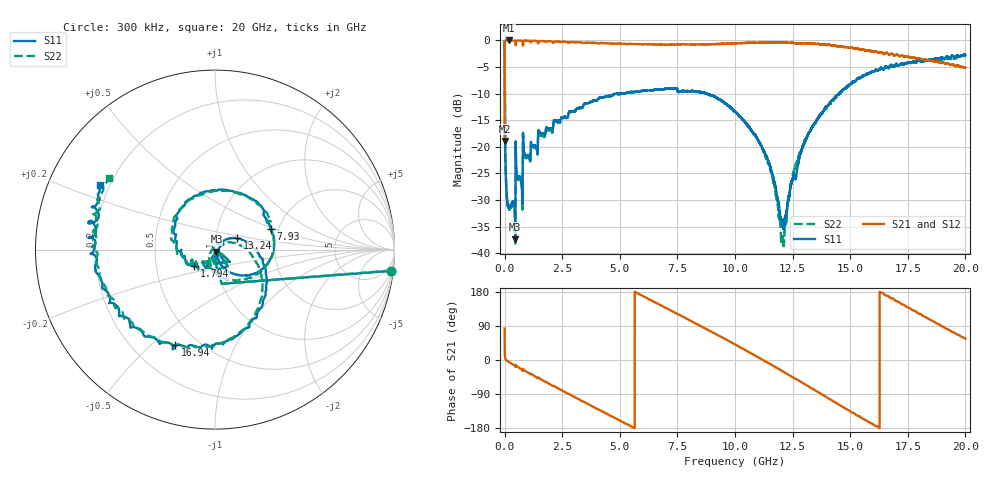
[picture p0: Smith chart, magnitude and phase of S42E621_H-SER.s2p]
!{S42E621}
!Johanson Technology Inc.
!www.johansontechnology.com
!Test Board Conditions:
!Substrate Type  RO4350B
!Substrate Thickness  50 mil
!Substrate Dk  3.66
!TL Type: GCPW
!TL Trace Width  60 mil
!TL Gap  10 mil
!Electrode orientation  Horizontal
!DUT TOPOLOGY	SERIES
!Mounting Pad LxW  14x55 mil
! Created Wed Nov 25 22:22:56 2020
# khz S ma R 50
! 2 Port Network Data from SP1.SP block
! freq  magS11  angS11  magS21  angS21  magS12  angS12  magS22  angS22
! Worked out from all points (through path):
!   20001 points, 300 kHz to 20 GHz, reference 50 ohm
!   highest |S21| = -0.01 dB at 192.3 MHz (marker M1); lowest = -18.9 dB at 300 kHz (marker M2)
!   group delay of S21, straight-line fit = 92.7 ps
!   lowest |S11| = -37.3 dB at 465.3 MHz (marker M3), VSWR 1.03, Z = 50.8 - j1.11 ohm
!   |S11| at or under -10 dB: 7.897 MHz to 4.985 GHz (4.977 GHz wide, 199 % of centre); 8.790778 GHz to 8.793084 GHz (2.307 MHz wide, 0.0262 % of centre); 8.796 GHz to 14.51 GHz (5.709 GHz wide, 49 % of centre)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
!   |S22| runs from -38.7 to -0.1 dB; largest |S21 - S12| = 0.016
!   S11 on the Smith chart (normalised r, x): 300 kHz: 2, -16; 1.794 GHz: 0.78, -0.15; 7.93 GHz: 1.83, +0.48; 13.24 GHz: 1.27, +0.17; 16.94 GHz: 0.38, -0.60; 20 GHz: 0.16, +0.26
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300  0.9872 -6.9  0.1138 82.9  0.1131 83.0  0.9896 -6.8
109300  0.03173 -89.7  0.9975 -2.3  0.9985 -2.3  0.0311 -89.8
192300  0.0271 -93.5  0.9984 -5.6  0.9969 -5.6  0.02615 -94.4
465300  0.01357 -53.3  0.9872 -16.9  0.9883 -16.9  0.01182 -46.6
887300  0.08346 -117.6  0.992 -28.2  0.9917 -28.2  0.07968 -117.8
1794300  0.1492 -141.3  0.9685 -57.7  0.9692 -57.7  0.1412 -144.5
3334300  0.2318 158.7  0.9554 -107.8  0.9564 -107.8  0.2306 168.0
5096300  0.3192 110.2  0.9312 -162.7  0.9325 -162.7  0.3154 107.8
6667300  0.346 61.9  0.915 147.8  0.9142 147.7  0.3449 56.3
7930300  0.3341 20.6  0.9193 108.0  0.92 108.0  0.3316 16.3
8977300  0.306 -14.0  0.9202 74.6  0.9208 74.6  0.3037 -15.7
1.00003e7  0.2154 -42.3  0.9372 41.1  0.9361 41.1  0.2145 -53.1
1.14133e7  0.07793 -70.1  0.951 -6.7  0.9496 -6.7  0.07202 -114.7
1.20693e7  0.01811 -20.9  0.9554 -29.8  0.9565 -29.9  0.01426 144.8
1.25873e7  0.05363 32.0  0.9386 -48.7  0.9386 -48.6  0.06145 40.2
1.32373e7  0.1388 27.4  0.9343 -71.3  0.9358 -71.3  0.1373 10.9
1.33343e7  0.1504 22.9  0.9333 -74.8  0.9332 -74.9  0.1503 7.5
1.50383e7  0.395 -47.6  0.8494 -137.0  0.8531 -136.9  0.3881 -50.0
1.66673e7  0.5492 -102.7  0.7374 168.0  0.7411 167.2  0.5641 -104.4
1.69383e7  0.576 -112.5  0.72 157.9  0.7311 157.5  0.5809 -113.2
1.84513e7  0.6634 -161.4  0.6487 106.6  0.6499 106.9  0.6462 -162.3
2e7  0.7328 150.6  0.5537 56.1  0.5541 56.5  0.7194 145.6
